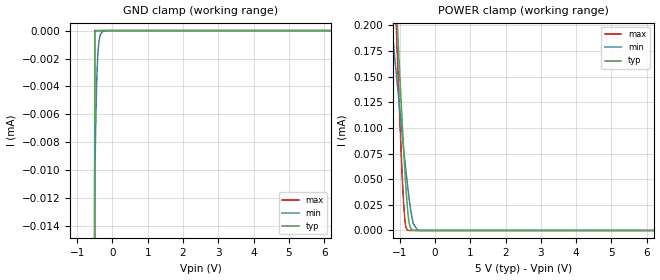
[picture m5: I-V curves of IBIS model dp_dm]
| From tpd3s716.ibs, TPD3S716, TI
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|   dp_dm Model
[Model]   dp_dm
Model_type   Terminator
|   typ   min   max
|   (nom PVT)   (fast PVT)   (slow PVT)
C_comp   1.403e-12   1.401e-12   1.577e-12
| Where nom  PVT is Nominal Process, 5V, 40C
|   Fast PVT is Strong Process,  5.5V, -40C
|   Slow PVT is Weak Process,   4.5V, 125C
[Voltage Range]   5   4.5   5.5
|Junction Temperature
[Temperature Range]   40   125   -40
[Power Clamp Reference]   5   4.5   5.5
[GND Clamp Reference]   0   0   0
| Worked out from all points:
|   GND clamp passes 1 mA (typ) near -1.11 V on its own axis
[GND Clamp]
|   Voltage   I(typ)   I(min)   I(max)
-5V       -546.3mA   -432.3mA   -725.9mA
-1.101V   -911.5uA   -945.4uA   -1.68mA
-500mV    -97.47nA   -11.01uA   0A
-482mV    -61.46nA   -7.793uA   0A
-464mV    -40.04nA   -5.361uA   0A
-446mV    -27.01nA   -3.591uA   0A
-423.5mV  -17.14nA   -2.115uA   0A
-401mV    -11.14nA   -1.222uA   0A
-374mV    0A         -625.1nA   0A
-338mV    0A         -255.1nA   0A
-288.5mV  0A         -77.6nA    0A
10V       0A         0A         0A
[POWER Clamp]
|   Voltage   I(typ)   I(min)   I(max)
-5V       3.26mA     1.664mA    4.19mA
-1.235V   322.9uA    203.3uA    331.9uA
-1.105V   227.4uA    155.6uA    206.9uA
-1.073V   204.4uA    144.1uA    177uA
-990mV    145.9uA    114.5uA    102.4uA
-891.5mV  80.66uA    80.45uA    27.8uA
-830mV    44.72uA    60.17uA    4.269uA
-770.5mV  17.77uA    41.72uA    284.2nA
-690mV    2.004uA    20.06uA    5.85nA
-621.5mV  181.9nA    7.22uA     0A
-464mV    0A         141.2nA    0A
10V       0A         0A         0A
